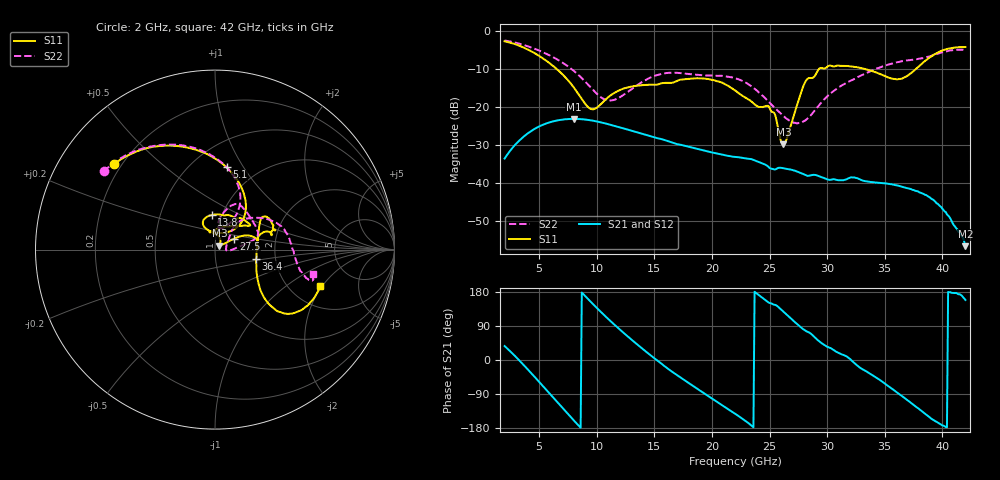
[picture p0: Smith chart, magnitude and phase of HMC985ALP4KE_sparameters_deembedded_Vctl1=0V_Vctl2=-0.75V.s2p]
!s2p File: Measurements: S11, S21, S12, S22
# GHz S dB R 50.0
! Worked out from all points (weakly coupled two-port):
!   401 points, 2 GHz to 42 GHz, reference 50 ohm
!   highest |S21| = -23.13 dB at 8 GHz (marker M1); lowest = -56.8 dB at 42 GHz (marker M2)
!   lowest |S11| = -29.8 dB at 26.2 GHz (marker M3), VSWR 1.07, Z = 52.4 + j2.25 ohm
!   |S11| at or under -10 dB: 6.541 GHz to 29.27 GHz (22.73 GHz wide, 127 % of centre); 33.34 GHz to 37.69 GHz (4.349 GHz wide, 12.2 % of centre)
!   |S22| runs from -24.3 to -2.4 dB; largest |S21 - S12| = 0.00017
!   S11 on the Smith chart (normalised r, x): 2 GHz: 0.17, +0.36; 5.1 GHz: 0.72, +0.84; 13.8 GHz: 0.90, +0.36; 27.5 GHz: 1.22, +0.15; 36.4 GHz: 1.58, -0.17; 42 GHz: 2.90, -1.91
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2  -2.64 139.9  -33.62 36.8  -33.63 36.8  -2.41 144.9
3.5  -4.09 112.1  -28.23 -8.2  -28.23 -8.2  -3.46 120.7
5.1  -6.69 82.0  -24.98 -61.3  -24.99 -61.3  -5.21 96.3
8  -14.80 45.4  -23.13 -159.2  -23.14 -159.2  -10.43 62.1
8.7  -17.90 51.7  -23.22 178.1  -23.22 178.1  -12.37 58.9
9.7  -20.59 86.2  -23.62 146.7  -23.63 146.7  -15.56 60.6
11  -17.39 114.7  -24.54 108.1  -24.54 108.1  -18.28 75.2
13.8  -14.27 95.3  -26.93 33.9  -26.93 33.8  -13.65 77.4
15.4  -13.94 73.0  -28.31 -4.6  -28.32 -4.6  -11.40 68.3
19.4  -12.52 34.6  -31.57 -89.6  -31.57 -89.6  -11.63 35.5
22  -15.59 52.2  -33.17 -141.5  -33.18 -141.5  -12.38 16.0
25  -20.20 97.8  -36.08 150.5  -36.09 150.5  -18.85 3.7
26.2  -29.81 41.4  -36.17 127.2  -36.18 127.2  -22.37 -4.9
27.5  -18.41 29.7  -37.16 91.7  -37.17 91.7  -24.24 3.6
28.1  -13.36 20.7  -37.96 77.4  -37.98 77.6  -23.54 17.6
28.7  -12.31 12.9  -37.97 66.3  -37.94 66.4  -21.73 30.7
31  -9.09 23.4  -39.35 18.5  -39.36 18.7  -14.79 50.9
33.3  -9.96 34.4  -39.59 -28.4  -39.60 -28.3  -11.20 39.8
35.4  -12.27 12.4  -40.32 -70.8  -40.33 -71.0  -8.72 24.6
36.4  -12.57 -12.8  -40.98 -93.2  -41.00 -93.2  -7.94 16.5
39.5  -5.80 -43.3  -45.43 -163.2  -45.38 -163.9  -6.00 -14.7
42  -4.14 -19.0  -56.76 158.5  -57.00 158.0  -4.96 -13.8
